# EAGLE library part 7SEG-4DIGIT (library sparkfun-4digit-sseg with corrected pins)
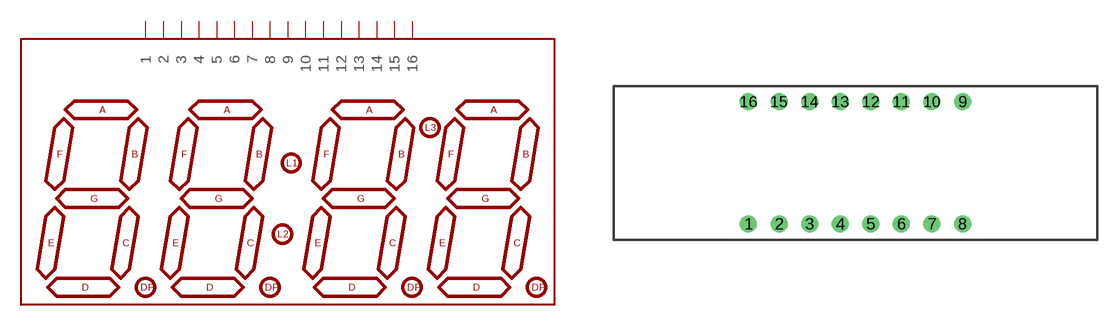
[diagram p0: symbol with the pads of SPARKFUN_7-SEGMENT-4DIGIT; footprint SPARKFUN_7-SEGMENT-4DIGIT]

Designator prefix -

## 7SEG-4DIGIT  [SPARKFUN_7-SEGMENT-4DIGIT]
1  1
2  2
3  3
4  4
5  5
6  6
7  7
8  8
9  9
10  10
11  11
12  12
13  13
14  14
15  15
16  16

## Footprint SPARKFUN_7-SEGMENT-4DIGIT (pad centres in mm)
drill 0.9: 1 -8.89,-5.08; 2 -6.35,-5.08; 3 -3.81,-5.08; 4 -1.27,-5.08; 5 1.27,-5.08; 6 3.81,-5.08; 7 6.35,-5.08; 8 8.89,-5.08; 9 8.89,5.08; 10 6.35,5.08; 11 3.81,5.08; 12 1.27,5.08; 13 -1.27,5.08; 14 -3.81,5.08; 15 -6.35,5.08; 16 -8.89,5.08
